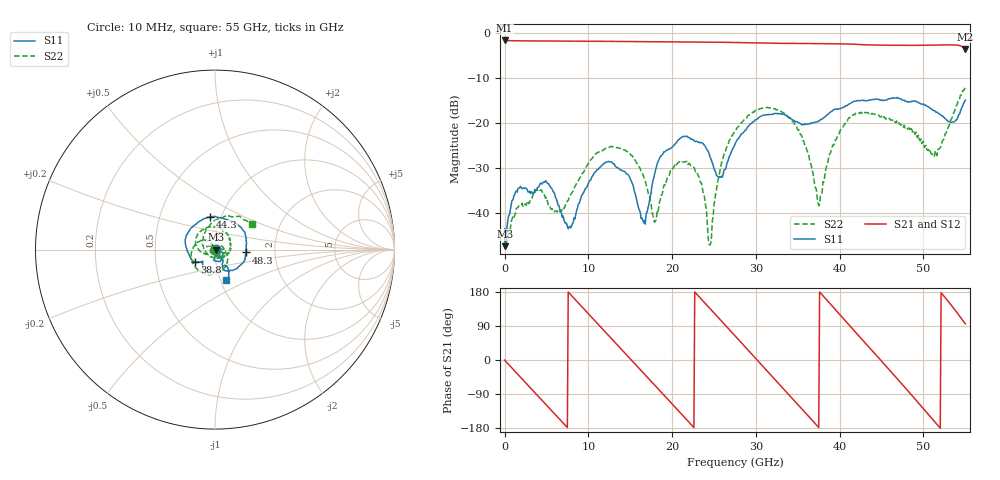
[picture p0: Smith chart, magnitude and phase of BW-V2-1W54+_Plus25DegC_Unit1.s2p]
!Mini-Circuits Laboratory
!S-Parameters
!Type: Fixed Attenuators
!Model: BW-V2-1W54+
!Run / Lot / Date Code: YE0105 / QN2150331 / 2150
!Fixture: N/A, Pressing Arm: N/A
!Network Analyzer: Keysight P9375A;  Serial number: 76634
!Date: 1/25/2022 at 8:22:08 AM
!S/N: Unit# 1 (U1 25°C)
!Tested with: 2 PORT CALIBRATION USING eCAL. DE-EMBEDDED 1.85MM F/F ADAPTER ON PORT 1. TEMP AT 25°C.
!Remark: UNITS TESTED IN 50 OHM SYSTEM, WITHOUT Z-CONVERSION, PORT EXTENSION OFF.
# Hz  S  dB  R  50
!Frequency  S11 dB  S11 Deg  S21 dB  S21 Deg  S12 dB  S12 Deg  S22 dB  S22 Deg
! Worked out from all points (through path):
!   559 points, 10 MHz to 55 GHz, reference 50 ohm
!   highest |S21| = -1.66 dB at 10 MHz (marker M1); lowest = -3.5 dB at 55 GHz (marker M2)
!   group delay of S21, straight-line fit = 67.3 ps
!   lowest |S11| = -47.3 dB at 100 MHz (marker M3), VSWR 1.01, Z = 50.4 - j0.035 ohm
!   |S11| at or under -10 dB: start of sweep to end of sweep
!   |S22| runs from -47.0 to -12.1 dB; largest |S21 - S12| = 0.0012
!   S11 on the Smith chart (normalised r, x): 10 MHz: 1.01, +0.00; 38.8 GHz: 0.79, -0.11; 44.3 GHz: 0.89, +0.33; 48.3 GHz: 1.42, -0.05; 55 GHz: 1.07, -0.37
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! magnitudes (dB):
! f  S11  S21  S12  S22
! 10 MHz  -44.8  -1.7  -1.7  -46.0
! 100 MHz  -47.3  -1.7  -1.7  -43.6
! 1.8 GHz  -34.3  -1.7  -1.7  -38.1
! 5.1 GHz  -33.3  -1.8  -1.8  -37.2
! 7.7 GHz  -43.1  -1.8  -1.8  -36.6
! 9.2 GHz  -36.0  -1.8  -1.8  -31.4
! 12.6 GHz  -28.6  -1.9  -1.9  -25.4
! 16.6 GHz  -42.1  -1.9  -1.9  -31.8
! 18.4 GHz  -28.2  -1.9  -1.9  -38.8
! 21.9 GHz  -23.2  -2.0  -2.0  -29.2
! 24.5 GHz  -27.5  -2.0  -2.0  -47.0
! 25.9 GHz  -31.8  -2.1  -2.1  -28.8
! 27.6 GHz  -24.3  -2.1  -2.1  -21.6
! 32.9 GHz  -17.9  -2.3  -2.3  -17.3
! 36.7 GHz  -20.0  -2.3  -2.3  -30.5
! 37.6 GHz  -19.4  -2.4  -2.4  -38.0
! 38.8 GHz  -17.7  -2.4  -2.4  -26.9
! 44.3 GHz  -14.7  -2.7  -2.7  -18.1
! 45.9 GHz  -14.6  -2.7  -2.7  -19.0
! 48.3 GHz  -15.2  -2.7  -2.7  -21.1
! 51.4 GHz  -17.3  -2.7  -2.7  -26.2
! 55 GHz  -14.9  -3.5  -3.5  -12.1
